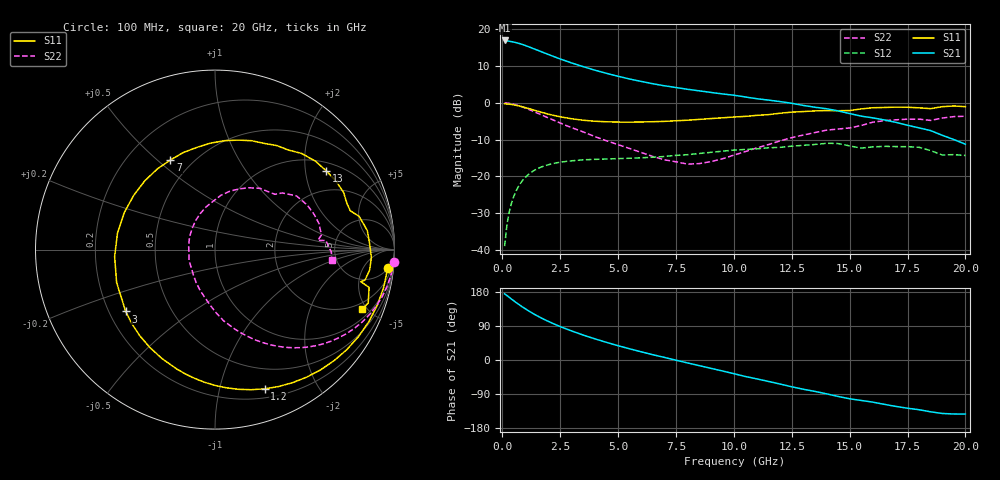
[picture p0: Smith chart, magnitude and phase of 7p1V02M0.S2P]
! Infineon Technologies  Discrete & RF Semiconductors
! bfp620
! VCE =  1.0 V,  IC =  2.0 mA
! Common Emitter S-Parameters:  Sep 2002
# GHz  S  MA  R  50
!  f  S11  S21  S12  S22
! GHz  MAG  ANG  MAG  ANG  MAG  ANG  MAG  ANG
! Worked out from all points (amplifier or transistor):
!   59 points, 100 MHz to 20 GHz, reference 50 ohm
!   highest |S21| = 16.9 dB at 100 MHz (marker M1)
!   |S21| within 3 dB of that: start of sweep to 1.661 GHz
!   unconditionally stable (mu >= 1): 5.852 GHz to 15.78 GHz; 17.25 GHz to end of sweep
!   at 1 GHz: K = 0.17, MSG = 17.9 dB, |S12| = -20.3 dB
!   at 5.5 GHz: K = 0.95, MSG = 10.8 dB, |S12| = -15.1 dB
!   at 20 GHz: K = 1.60, MAG = -3.0 dB, |S12| = -14.3 dB
!   S11 on the Smith chart (normalised r, x): 100 MHz: 5, -17; 1.2 GHz: 0.29, -1.38; 3 GHz: 0.27, -0.29; 7 GHz: 0.38, +0.55; 13 GHz: 1.25, +2.59; 20 GHz: 1.51, -4.65
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0.1  0.9676 -6.2  7.037 174.6  0.0112 83.8  0.9972 -4.0
0.3  0.9562 -18.8  6.872 165.4  0.0327 79.6  0.9817 -11.8
0.5  0.9354 -31.1  6.679 156.0  0.0536 72.2  0.9525 -19.2
0.7  0.9075 -42.9  6.439 147.2  0.0727 64.9  0.9139 -26.2
0.9  0.8751 -54.3  6.152 138.8  0.0895 58.1  0.8693 -32.6
1.2  0.8234 -70.4  5.679 127.3  0.1102 48.9  0.7975 -41.3
1.6  0.7566 -90.0  5.069 113.6  0.1303 38.7  0.7034 -51.0
2  0.699 -107.6  4.525 101.6  0.144 30.4  0.6201 -59.2
2.4  0.6548 -123.8  4.048 90.8  0.1535 23.5  0.5478 -66.3
3  0.6053 -145.3  3.472 76.5  0.1624 15.0  0.4581 -75.8
3.5  0.5781 -161.5  3.095 65.7  0.1675 9.2  0.4005 -83.0
4  0.5605 -176.0  2.773 55.8  0.1698 4.2  0.3465 -89.8
5  0.546 157.8  2.291 37.7  0.1739 -3.0  0.2692 -102.8
6  0.5477 135.5  1.951 21.6  0.1786 -8.8  0.2107 -120.1
7  0.5579 116.4  1.701 6.9  0.1859 -13.3  0.1677 -141.3
8.5  0.5937 92.4  1.453 -14.8  0.204 -21.1  0.1487 171.0
10.5  0.6528 64.9  1.198 -43.6  0.2319 -35.6  0.2168 112.4
13  0.7589 35.5  0.92 -77.1  0.2638 -54.5  0.364 68.3
13.5  0.7746 29.7  0.869 -82.9  0.2708 -59.2  0.393 61.2
15  0.7842 16.0  0.713 -102.3  0.2592 -79.1  0.4545 42.7
17  0.8724 -2.9  0.541 -122.5  0.2536 -90.6  0.5864 19.5
20  0.8849 -22.1  0.273 -142.6  0.1918 -111.6  0.6557 -5.3
